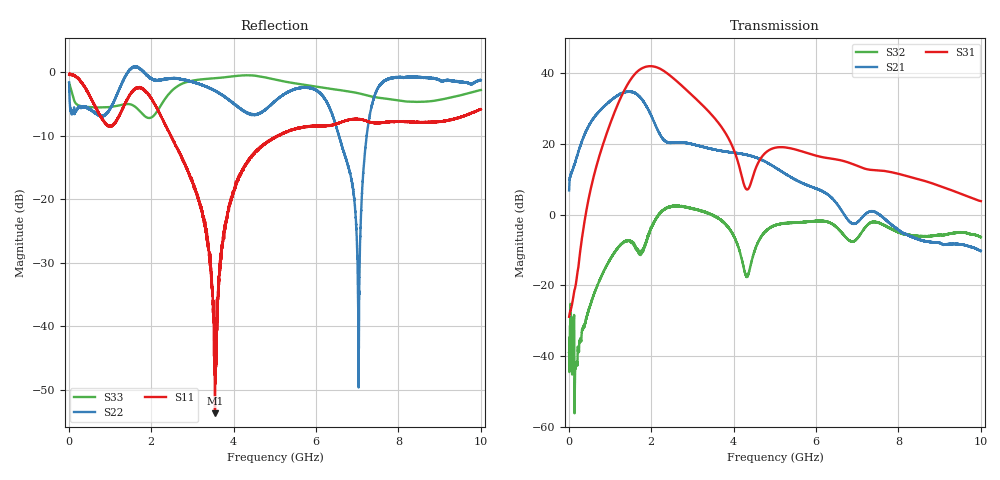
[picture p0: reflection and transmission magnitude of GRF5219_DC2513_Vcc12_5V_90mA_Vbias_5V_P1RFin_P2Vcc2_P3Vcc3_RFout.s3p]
!Keysight Technologies,N5245B,MY56052315,A.20.20.05
!Date: Friday, August 21, 2026 15:37:09
!Correction: S11(C  3-Port  )
!S12(C  3-Port  )
!S13(C  3-Port  )
!S21(C  3-Port  )
!S22(C  3-Port  )
!S23(C  3-Port  )
!S31(C  3-Port  )
!S32(C  3-Port  )
!S33(C  3-Port  )
!S3P File: Measurements: <S11,S12,S13>,
!<S21,S22,S23>,
!<S31,S32,S33>:
# Hz S  dB  R 50
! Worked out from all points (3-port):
!   9991 points, 10 MHz to 10 GHz, reference 50 ohm
!   strongest paths, dB at 10 MHz, 2.507 GHz, 5.005 GHz, 7.503 GHz, 10 GHz:
!     S31: -28.9, 38.9, 18.9, 12.6, 3.8
!     S21: 6.9, 20.3, 13.4, 0.3, -10.3
!     S32: -38.9, 2.3, -3.0, -2.2, -6.4
!   lowest |S11| = -53.8 dB at 3.549 GHz (marker M1), VSWR 1.00, Z = 50 - j0.204 ohm
!   |S11| at or under -10 dB: 2.482 GHz to 5.066 GHz (2.583 GHz wide, 68.5 % of centre); 5.066144 GHz to 5.070442 GHz (4.299 MHz wide, 0.0848 % of centre); 5.071299 GHz to 5.075143 GHz (3.844 MHz wide, 0.0758 % of centre)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
1e7  -0.38 -1.9  -58.89 106.7  -51.11 -26.8
     6.85 70.4  -1.59 -56.0  -52.53 -77.0
     -28.91 -175.5  -38.94 16.3  -1.66 -57.0
6.76e8  -5.79 -99.1  -40.32 105.4  -67.00 103.4
        28.43 24.7  -6.52 169.8  -39.89 -66.6
        13.87 5.0  -20.61 -1.0  -5.54 -172.1
1.185e9  -7.42 -109.7  -37.45 86.1  -61.60 91.6
         33.72 -33.9  -3.34 -162.1  -29.54 -137.2
         31.06 -59.3  -9.51 -74.2  -5.28 -174.1
1.526e9  -3.16 -142.4  -34.60 90.1  -56.60 91.3
         34.75 -88.6  0.66 179.9  -25.95 161.6
         38.63 -125.1  -7.91 -158.5  -5.11 -179.5
1.842e9  -2.84 166.2  -32.65 77.2  -55.23 59.1
         31.50 -143.0  -0.11 153.1  -28.42 109.6
         41.74 166.9  -9.00 40.1  -6.90 -178.0
2.187e9  -6.28 117.9  -33.19 70.8  -54.90 50.0
         23.26 -170.0  -1.30 142.6  -33.00 107.8
         41.46 99.7  0.15 -67.5  -5.74 -157.9
2.617e9  -11.80 75.8  -33.05 80.4  -58.64 58.0
         20.46 -154.5  -0.99 130.4  -29.65 95.5
         37.82 34.5  2.36 -143.4  -2.30 -164.9
3.549e9  -53.75 -83.2  -28.52 89.2  -55.00 57.6
         18.42 175.5  -2.89 127.9  -30.38 37.1
         27.19 -58.3  -0.36 125.3  -0.93 168.7
5.005e9  -10.33 152.7  -27.20 64.5  -53.04 95.6
         13.39 107.6  -4.57 117.2  -39.26 54.5
         18.93 -38.0  -2.98 134.0  -1.15 148.0
1e10  -5.81 103.3  -25.74 36.0  -56.71 15.4
      -10.27 57.4  -1.24 86.4  -29.51 -16.7
      3.83 124.8  -6.41 -37.5  -2.80 75.7
